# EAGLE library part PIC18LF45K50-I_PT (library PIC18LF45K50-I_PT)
Microchip PIC18LF45K50-I/PT, 8bit PIC Microcontroller, 48MHz, 32 kB Flash, 44-Pin TQFP Source: Datasheet
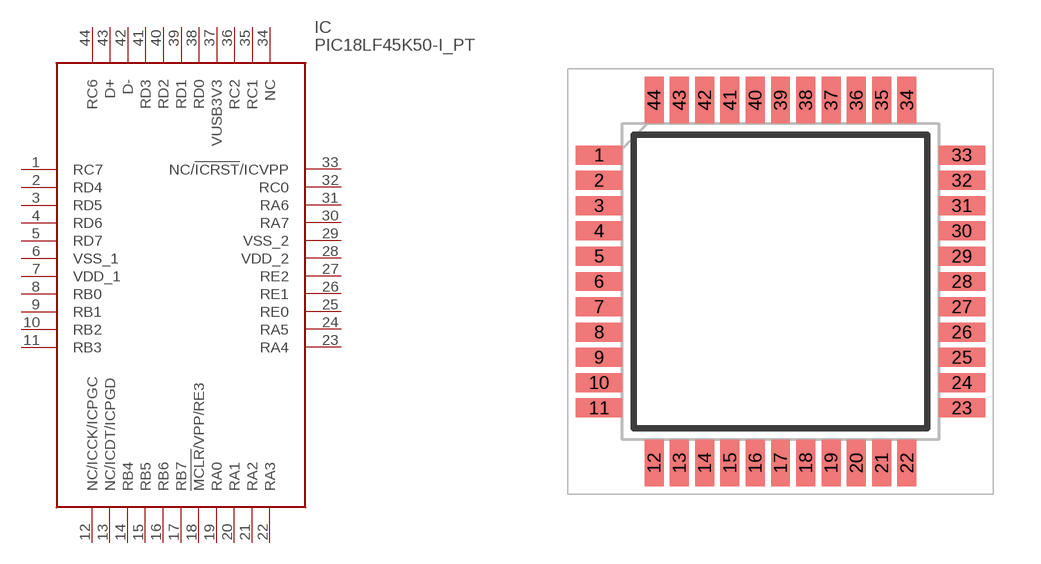
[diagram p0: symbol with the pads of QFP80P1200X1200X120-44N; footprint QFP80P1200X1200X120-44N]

Designator prefix IC

## PIC18LF45K50-I_PT (Description: Microchip PIC18LF45K50-I/PT, 8bit PIC Microcontroller, 48MHz, 32 kB Flash, 44-Pin TQFP; Height: 1.2mm; Manufacturer_Name: Microchip; Manufacturer_Part_Number: PIC18LF45K50-I/PT; Mouser_Part_Number: 579-PIC18LF45K50I/PT; Mouser_Price-Stock: https://www.mouser.com/Search/Refine.aspx?Keyword=579-PIC18LF45K50I%2FPT)  [QFP80P1200X1200X120-44N]
1  RC7
2  RD4
3  RD5
4  RD6
5  RD7
6  VSS_1
7  VDD_1
8  RB0
9  RB1
10  RB2
11  RB3
12  NC/ICCK/ICPGC
13  NC/ICDT/ICPGD
14  RB4
15  RB5
16  RB6
17  RB7
18  !MCLR!/VPP/RE3
19  RA0
20  RA1
21  RA2
22  RA3
23  RA4
24  RA5
25  RE0
26  RE1
27  RE2
28  VDD_2
29  VSS_2
30  RA7
31  RA6
32  RC0
33  NC/!ICRST!/ICVPP
34  NC  nc
35  RC1
36  RC2
37  VUSB3V3
38  RD0
39  RD1
40  RD2
41  RD3
42  D-
43  D+
44  RC6

## Footprint QFP80P1200X1200X120-44N (pad centres in mm)
44-Lead 10x10x1 mm Body 2.00mm TQFP
smd 1.475 x 0.6: 1 -5.738,4; 2 -5.738,3.2; 3 -5.738,2.4; 4 -5.738,1.6; 5 -5.738,0.8; 6 -5.738,0; 7 -5.738,-0.8; 8 -5.738,-1.6; 9 -5.738,-2.4; 10 -5.738,-3.2; 11 -5.738,-4; 23 5.738,-4; 24 5.738,-3.2; 25 5.738,-2.4; 26 5.738,-1.6; 27 5.738,-0.8; 28 5.738,0; 29 5.738,0.8; 30 5.738,1.6; 31 5.738,2.4; 32 5.738,3.2; 33 5.738,4
smd 0.6 x 1.475: 12 -4,-5.738; 13 -3.2,-5.738; 14 -2.4,-5.738; 15 -1.6,-5.738; 16 -0.8,-5.738; 17 0,-5.738; 18 0.8,-5.738; 19 1.6,-5.738; 20 2.4,-5.738; 21 3.2,-5.738; 22 4,-5.738; 34 4,5.738; 35 3.2,5.738; 36 2.4,5.738; 37 1.6,5.738; 38 0.8,5.738; 39 0,5.738; 40 -0.8,5.738; 41 -1.6,5.738; 42 -2.4,5.738; 43 -3.2,5.738; 44 -4,5.738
